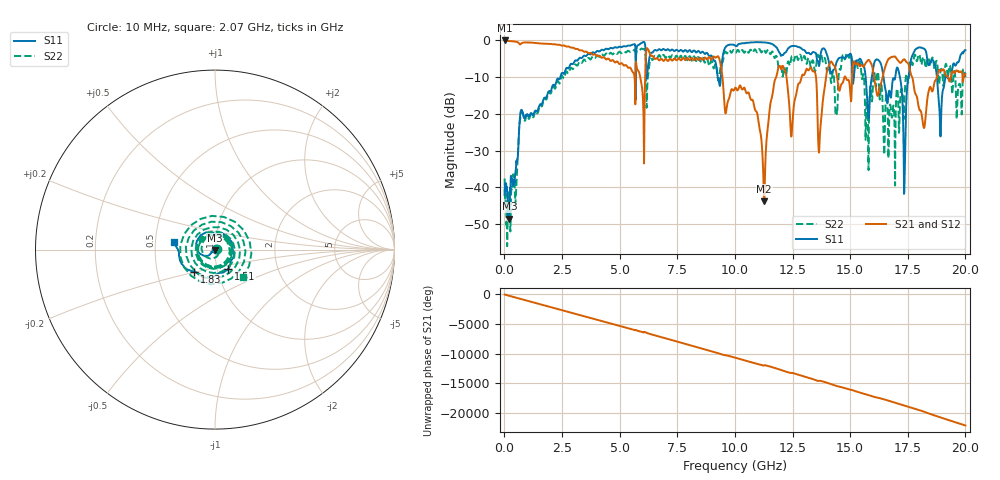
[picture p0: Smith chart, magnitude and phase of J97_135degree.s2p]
!Keysight Technologies,N5222A,MY51421036,A.10.65.16
!Date: Friday, March 31, 2023 15:12:15
!Correction: S11(Full 2 Port(1,2))
!S21(Full 2 Port(1,2))
!S12(Full 2 Port(1,2))
!S22(Full 2 Port(1,2))
!S2P File: Measurements: S11, S21, S12, S22:
# Hz S  dB  R 50
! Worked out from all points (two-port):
!   2000 points, 10 MHz to 20 GHz, reference 50 ohm
!   highest |S21| = -0.04 dB at 10 MHz (marker M1); lowest = -43.8 dB at 11.27 GHz (marker M2)
!   |S21| within 3 dB of the highest: start of sweep to 3.429 GHz; 6.153 GHz to 6.278 GHz (124.9 MHz wide, 2.01 % of centre)
!   lowest |S11| = -48.5 dB at 220 MHz (marker M3), VSWR 1.01, Z = 49.8 - j0.332 ohm
!   |S11| at or under -10 dB: start of sweep to 2.43 GHz; 16.45 GHz to 16.96 GHz (510.8 MHz wide, 3.06 % of centre); 18.76 GHz to 19.14 GHz (375.6 MHz wide, 1.98 % of centre)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
!   |S22| runs from -56.0 to -2.2 dB; largest |S21 - S12| = 0.014
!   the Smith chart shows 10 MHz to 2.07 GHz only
!   S11 on the Smith chart (normalised r, x): 10 MHz: 1.01, +0.01; 1.51 GHz: 1.13, -0.24; 1.83 GHz: 0.77, -0.19; 2.07 GHz: 0.63, +0.06
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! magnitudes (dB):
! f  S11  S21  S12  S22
! 10 MHz  -42.0  0.0  -0.1  -37.6
! 220 MHz  -48.5  -0.2  -0.2  -41.3
! 730 MHz  -19.1  -0.9  -0.9  -20.2
! 1.51 GHz  -17.8  -0.8  -0.8  -18.1
! 1.83 GHz  -15.4  -0.9  -0.9  -16.0
! 2.07 GHz  -12.7  -1.0  -1.0  -13.2
! 3.35 GHz  -4.8  -2.7  -2.7  -6.2
! 6.68 GHz  -2.5  -5.3  -5.3  -4.2
! 10.01 GHz  -1.4  -13.0  -12.9  -3.2
! 11.27 GHz  -0.6  -43.8  -44.1  -2.5
! 11.89 GHz  -2.9  -7.4  -7.3  -7.3
! 12.46 GHz  -1.6  -25.8  -25.8  -4.4
! 13.34 GHz  -3.5  -7.9  -7.9  -5.9
! 13.68 GHz  -5.8  -26.7  -26.7  -4.2
! 14.13 GHz  -8.1  -6.2  -6.1  -9.0
! 16.67 GHz  -14.4  -5.1  -5.0  -29.1
! 17.1 GHz  -8.3  -5.7  -5.6  -19.8
! 17.36 GHz  -38.2  -5.2  -5.2  -16.0
! 17.66 GHz  -4.8  -9.7  -9.6  -5.7
! 18.18 GHz  -2.2  -23.4  -23.5  -4.5
! 18.91 GHz  -25.1  -8.2  -8.1  -8.8
! 20 GHz  -2.7  -9.1  -9.1  -10.1
